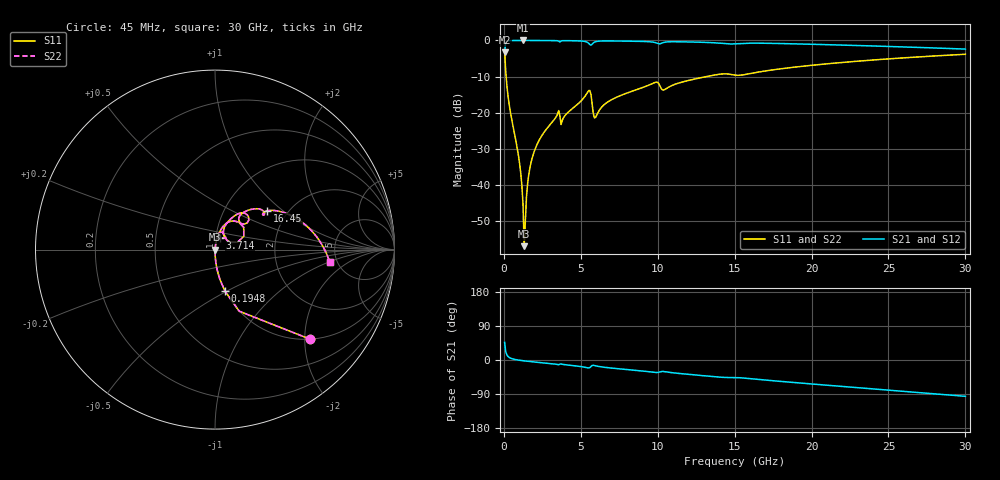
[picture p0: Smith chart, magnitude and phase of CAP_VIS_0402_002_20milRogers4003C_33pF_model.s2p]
! S-parameter model data by Modelithics Inc.  support@modelithics.com  813-866-6335  Tampa FL USA
! S-Parameter data specifications:
! Substrate: 20-mil Rogers 4003C, substrate thickness, H=0.508mm, Dielectric constant, Er=3.75
! PCB Mounting Pad Footprint: Pad width, PadW=0.50mm , Pad length, PadL=0.50mm , Pad gap, PadG (edge-to-edge)=0.40mm , Reference planes=1.4mm apart
! Created Wed Nov 18 12:54:17 2015
# hz S ma R 50
! 2 Port Network Data from SP1.SP block
! freq  magS11  angS11  magS21  angS21  magS12  angS12  magS22  angS22
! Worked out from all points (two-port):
!   401 points, 45 MHz to 30 GHz, reference 50 ohm
!   highest |S21| = -0.01 dB at 1.243 GHz (marker M1); lowest = -3.3 dB at 45 MHz (marker M2)
!   |S21| within 3 dB of the highest: 53.13 MHz to end of sweep
!   lowest |S11| = -57.0 dB at 1.318 GHz (marker M3), VSWR 1.00, Z = 50.1 - j0.104 ohm
!   |S11| at or under -10 dB: 145.4 MHz to 13.18 GHz (13.03 GHz wide, 196 % of centre)
!   |S22| runs from -57.0 to -2.7 dB; largest |S21 - S12| = 0
!   S11 on the Smith chart (normalised r, x): 45 MHz: 1.00, -2.13; 194.8 MHz: 1.00, -0.48; 3.714 GHz: 1.05, +0.13; 16.45 GHz: 1.58, +0.78; 30 GHz: 4.34, -1.05
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4.5e7  0.7292 -43.2  0.6841 46.7  0.6841 46.7  0.7292 -43.2
1.94775e8  0.2345 -76.7  0.9717 13.2  0.9717 13.2  0.2345 -76.7
3.4455e8  0.129 -83.0  0.9911 6.8  0.9911 6.8  0.129 -83.0
1.018538e9  0.01983 -88.1  0.9989 -0.7  0.9989 -0.7  0.01983 -88.1
1.2432e9  0.005315 -81.3  0.999 -1.9  0.999 -1.9  0.005315 -81.3
1.318088e9  0.001418 -46.9  0.9989 -2.3  0.9989 -2.3  0.001418 -46.9
1.467862e9  0.006888 78.1  0.9989 -3.0  0.9989 -3.0  0.006888 78.1
1.692525e9  0.01735 82.2  0.9987 -4.1  0.9987 -4.1  0.01735 82.2
2.066962e9  0.03292 82.2  0.9981 -5.6  0.9981 -5.6  0.03292 82.2
3.414938e9  0.08892 76.2  0.992 -11.3  0.992 -11.3  0.08892 76.2
3.714488e9  0.06852 67.0  0.9829 -10.5  0.9829 -10.5  0.06852 67.0
5.062462e9  0.1486 68.9  0.9799 -17.7  0.9799 -17.7  0.1486 68.9
5.511788e9  0.2023 49.0  0.9122 -20.9  0.9122 -20.9  0.2023 49.0
5.961112e9  0.08634 50.7  0.9615 -15.3  0.9615 -15.3  0.08634 50.7
7.2342e9  0.1603 65.9  0.9819 -22.3  0.9819 -22.3  0.1603 65.9
1.007992e10  0.2498 41.1  0.8982 -32.0  0.8982 -32.0  0.2498 41.1
1.045436e10  0.2088 50.1  0.9451 -30.8  0.9451 -30.8  0.2088 50.1
1.50225e10  0.3307 35.4  0.8963 -46.3  0.8963 -46.3  0.3307 35.4
1.644536e10  0.3615 36.6  0.9166 -51.0  0.9166 -51.0  0.3615 36.6
2.003996e10  0.4532 25.8  0.8844 -63.4  0.8844 -63.4  0.4532 25.8
2.505742e10  0.5563 9.7  0.8246 -79.8  0.8246 -79.8  0.5563 9.7
3e10  0.6433 -6.3  0.7589 -95.9  0.7589 -95.9  0.6433 -6.3
